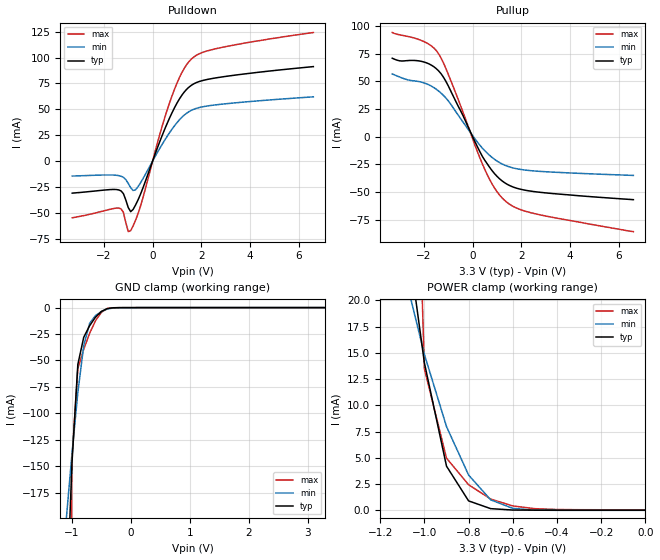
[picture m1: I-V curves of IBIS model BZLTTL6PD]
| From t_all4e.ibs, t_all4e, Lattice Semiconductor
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|   BZLTTL6PD
[Model]   BZLTTL6PD
Model_type   I/O
Polarity   Non-Inverting
Enable   Active-Low
C_comp   2pF   2pF   2pF
Vinl = 0.5
Vinh = 2.64
[Temperature Range]   25.0000   125.0000   -40.0000
[Voltage Range]   3.3000V   3.0000V   3.6000V
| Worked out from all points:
|   slope of the pulldown table from 0 to 0.495 V, typ, clamps not added: 16.1 ohm
|   slope of the pullup table from 0 to 0.495 V, typ, clamps not added: 23.4 ohm
|   GND clamp passes 1 mA (typ) near -0.40 V on its own axis
|   POWER clamp passes 1 mA (typ) near -0.80 V on its own axis
[Pulldown]
|voltage   I(typ)   I(min)   I(max)
-3.3V     -30.88mA   -14.4mA    -54.7mA
-1.4V     -27.72mA   -13.92mA   -45.3mA
-1.2V     -31.29mA   -15.59mA   -49.39mA
-1V       -44.8mA    -21.51mA   -68.08mA
-900mV    -48.78mA   -25.66mA   -67.21mA
-600mV    -37.58mA   -24.7mA    -50.92mA
300mV     19.17mA    12.56mA    26.25mA
800mV     46.84mA    30.97mA    63.2mA
1.3V      66.75mA    44.48mA    89.65mA
1.7V      74.79mA    50.19mA    100.7mA
3V        81.83mA    55.4mA     110.6mA
6.6V      91.29mA    62.1mA     124.2mA
[Pullup]
|voltage   I(typ)   I(min)   I(max)
-3.3V     70.9mA     56.74mA    94.14mA
-2V       67.51mA    48.64mA    85.98mA
-1.6V     63.33mA    44.48mA    80.35mA
-1.4V     59.56mA    41.33mA    75.01mA
-1.1V     50.13mA    35.01mA    61.78mA
-800mV    36.81mA    26.18mA    45.38mA
500mV     -21.4mA    -12.69mA   -29.67mA
900mV     -33.46mA   -20.53mA   -46.48mA
1.4V      -42.83mA   -26.51mA   -59.26mA
1.9V      -47.19mA   -29.39mA   -65.44mA
2.6V      -49.89mA   -31.15mA   -69.9mA
6.6V      -56.99mA   -35.07mA   -85.9mA
[GND_clamp]
|voltage   I(typ)   I(min)   I(max)
-3.3V     -4.405A    -1.803A    -40.47A
-1.1V     -296.4mA   -202.8mA   -979.3mA
-1V       -147.6mA   -138.6mA   -143.7mA
-900mV    -53.79mA   -80.42mA   -57.6mA
-800mV    -28.05mA   -35.98mA   -39.41mA
-700mV    -17.1mA    -14.8mA    -24.33mA
-600mV    -8.999mA   -7.523mA   -12.36mA
-500mV    -3.595mA   -3.617mA   -4.359mA
-400mV    -879.9uA   -1.324mA   -818.8uA
-300mV    -134.5uA   -303.4uA   -113.2uA
3.3V      27.16uA    10.44uA    65.22uA
[POWER_clamp]
|voltage   I(typ)   I(min)   I(max)
-3.3V     682mA      379.6mA    3.878A
-1.1V     29.47mA    23.43mA    82.94mA
-1V       14.05mA    14.85mA    13.46mA
-900mV    4.218mA    7.985mA    4.978mA
-800mV    910uA      3.369mA    2.448mA
-700mV    172.8uA    1.011mA    1.084mA
-600mV    39.84uA    197.6uA    429.9uA
-500mV    27.92uA    30.49uA    170.3uA
-400mV    27.27uA    11.82uA    89.74uA
0V        27.16uA    10.3uA     65.38uA
[Ramp]
| variable   typ   min   max
dV/dt_r   1.2315/1.0200ns   0.8308/2.3607ns   1.5922/0.3789ns
dV/dt_f   1.4788/1.1048ns   1.1687/2.4507ns   1.7342/0.5175ns
